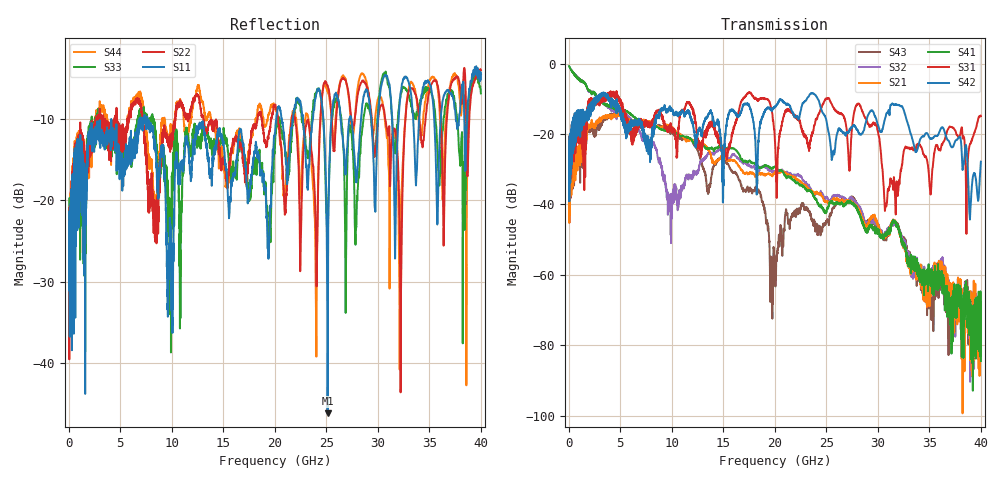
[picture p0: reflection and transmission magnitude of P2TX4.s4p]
!Agilent Technologies,N5245A,MY49151084,A.09.20.08
!Agilent N5245A: A.09.20.08
!Date: Thursday, March 01, 2012 10:55:16
!Correction: S11(Full 4 Port(1,2,3,4))
!S12(Full 4 Port(1,2,3,4))
!S13(Full 4 Port(1,2,3,4))
!S14(Full 4 Port(1,2,3,4))
!S21(Full 4 Port(1,2,3,4))
!S22(Full 4 Port(1,2,3,4))
!S23(Full 4 Port(1,2,3,4))
!S24(Full 4 Port(1,2,3,4))
!S31(Full 4 Port(1,2,3,4))
!S32(Full 4 Port(1,2,3,4))
!S33(Full 4 Port(1,2,3,4))
!S34(Full 4 Port(1,2,3,4))
!S41(Full 4 Port(1,2,3,4))
!S42(Full 4 Port(1,2,3,4))
!S43(Full 4 Port(1,2,3,4))
!S44(Full 4 Port(1,2,3,4))
!S4P File: Measurements: <S11,S12,S13,S14>,
!<S21,S22,S23,S24>,
!<S31,S32,S33,S34>,
!<S41,S42,S43,S44>:
# Hz S  dB  R 50
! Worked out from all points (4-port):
!   3996 points, 50 MHz to 40 GHz, reference 50 ohm
!   strongest paths, dB at 50 MHz, 10.04 GHz, 20.03 GHz, 30.02 GHz, 40 GHz:
!     S42: -24.9, -13.2, -12.4, -17.4, -27.9
!     S31: -24.8, -19.7, -22.3, -19.4, -14.9
!     S41: -0.8, -19.3, -29.2, -47.7, -84.5
!     S21: -41.8, -18.0, -30.8, -46.1, -65.2
!     S32: -0.8, -37.2, -30.7, -46.0, -78.7
!     S43: -42.5, -19.6, -59.7, -46.9, -71.0
!   lowest |S11| = -46.2 dB at 25.13 GHz (marker M1), VSWR 1.01, Z = 50.3 + j0.419 ohm
!   |S11| at or under -10 dB: start of sweep to 4.14 GHz; 4.142 GHz to 6.87 GHz (2.728 GHz wide, 49.6 % of centre); 7.635 GHz to 20.14 GHz (12.51 GHz wide, 90.1 % of centre)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
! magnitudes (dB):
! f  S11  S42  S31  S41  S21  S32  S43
! 50 MHz  -24.1  -24.9  -24.8  -0.8  -41.8  -0.8  -42.5
! 4.85 GHz  -14.8  -13.3  -10.5  -13.0  -14.3  -13.9  -14.4
! 9.82 GHz  -22.1  -12.1  -18.0  -19.1  -18.0  -39.9  -19.5
! 19.68 GHz  -16.9  -13.3  -13.3  -29.8  -31.5  -30.7  -56.4
! 25.13 GHz  -46.2  -18.1  -9.9  -40.9  -39.2  -38.1  -44.7
! 30.78 GHz  -4.5  -14.8  -39.8  -48.0  -48.7  -47.9  -49.4
! 40 GHz  -5.1  -27.9  -14.9  -84.5  -65.2  -78.7  -71.0
